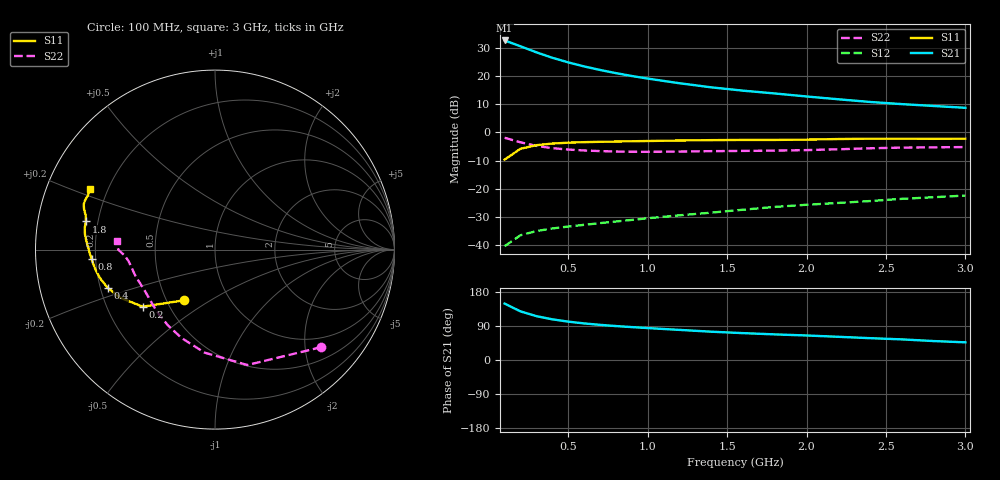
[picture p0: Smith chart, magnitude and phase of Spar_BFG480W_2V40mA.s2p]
! Filename: 240BFG480.001
! Title: BFG480W
! Bias: Vce=2V; Ic=40mA
! Company: NXP Semiconductors NL
! User: Quality&Reliability T&D
! Measure time: 10 Nov 1999 / 11:53:50
#  MHz  S  MA  R 50
! Freq  S11  S21  S12  S22  :
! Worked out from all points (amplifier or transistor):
!   20 points, 100 MHz to 3 GHz, reference 50 ohm
!   highest |S21| = 32.5 dB at 100 MHz (marker M1)
!   |S21| within 3 dB of that: start of sweep to 243.8 MHz
!   unconditionally stable (mu >= 1): 1.033 GHz to end of sweep
!   at 400 MHz: K = 0.59, MSG = 30.2 dB, |S12| = -34.0 dB
!   at 1.2 GHz: K = 1.04, MAG = 22.1 dB, |S12| = -29.3 dB
!   at 3 GHz: K = 1.12, MAG = 13.4 dB, |S12| = -22.3 dB
!   S11 on the Smith chart (normalised r, x): 100 MHz: 0.61, -0.39; 200 MHz: 0.36, -0.31; 400 MHz: 0.23, -0.16; 800 MHz: 0.18, -0.04; 1.8 GHz: 0.15, +0.11; 3 GHz: 0.13, +0.23
100  0.3305 -121.3  42.35 148.8  0.009705 67.0  0.8038 -42.5
200  0.5131 -141.7  33.39 128.3  0.01515 54.2  0.6679 -74.3
300  0.5941 -153.3  26.11 115.7  0.01796 49.3  0.5769 -95.8
400  0.6345 -160.4  20.93 107.3  0.01995 48.1  0.5263 -110.8
500  0.6579 -165.6  17.36 101.2  0.02159 48.8  0.4972 -121.7
600  0.672 -169.5  14.71 96.5  0.02314 50.0  0.4791 -129.8
700  0.6814 -172.7  12.74 92.8  0.02479 51.9  0.467 -136.1
800  0.689 -175.5  11.2 89.6  0.02653 53.7  0.4591 -141.3
900  0.6973 -177.9  9.957 86.9  0.02827 55.9  0.4547 -145.7
1000  0.7042 179.8  8.966 84.3  0.03024 57.4  0.4535 -149.6
1200  0.7189 176.1  7.411 79.5  0.03411 60.2  0.458 -156.0
1400  0.7298 173.2  6.277 74.7  0.03804 62.4  0.4658 -160.8
1600  0.7359 170.5  5.48 70.9  0.04283 64.3  0.4705 -164.6
1800  0.7361 167.7  4.886 67.6  0.04804 65.8  0.476 -168.3
2000  0.7451 165.2  4.323 64.7  0.05244 67.1  0.4862 -172.5
2200  0.7634 162.9  3.856 61.2  0.05648 67.8  0.503 -176.0
2400  0.7739 160.9  3.458 57.6  0.06101 67.9  0.5237 -178.4
2600  0.7742 159.1  3.166 54.4  0.06678 67.8  0.5383 -179.9
2800  0.7695 156.7  2.935 50.0  0.07129 66.8  0.5441 178.1
3000  0.7737 154.0  2.725 46.6  0.07638 66.5  0.5506 175.2
